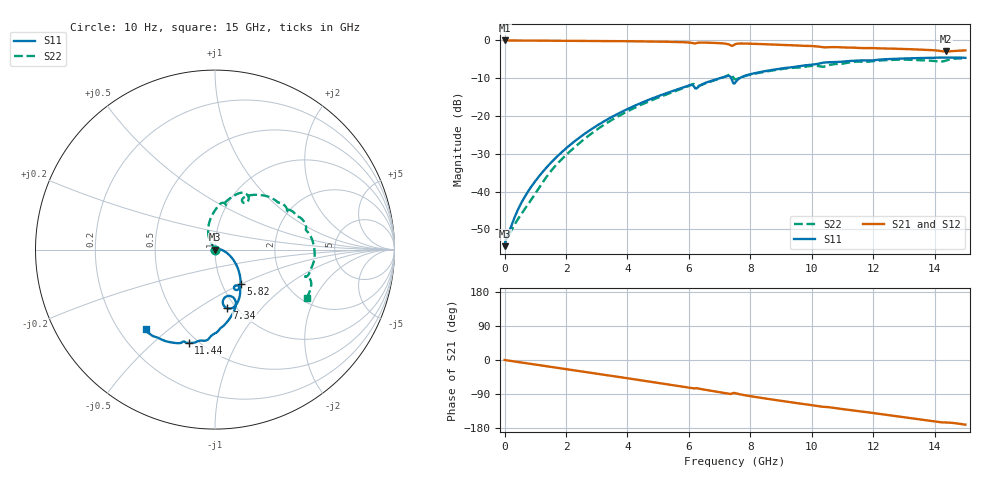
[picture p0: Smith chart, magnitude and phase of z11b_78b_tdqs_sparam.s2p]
![Disclaimer] This software code/ model/ data and all associated documentation, comments
!    or other information (collectively "Software") is provided
!    "AS IS" without warranty of any kind. MICRON TECHNOLOGY, INC.
!   ("MTI") EXPRESSLY DISCLAIMS ALL WARRANTIES EXPRESS OR IMPLIED,
!    INCLUDING BUT NOT LIMITED TO, NONINFRINGEMENT OF THIRD PARTY
!   RIGHTS, AND ANY IMPLIED WARRANTIES OF MERCHANTABILITY OR FITNESS
!    FOR ANY PARTICULAR PURPOSE. MTI DOES NOT WARRANT THAT THE
!    SOFTWARE WILL MEET YOUR REQUIREMENTS, OR THAT THE OPERATION OF
!    THE SOFTWARE WILL BE UNINTERRUPTED OR ERROR-FREE. FURTHERMORE,
!    MTI DOES NOT MAKE ANY REPRESENTATIONS REGARDING THE USE OR THE
!    RESULTS OF THE USE OF THE SOFTWARE IN TERMS OF ITS CORRECTNESS,
!    ACCURACY, RELIABILITY, OR OTHERWISE. THE ENTIRE RISK ARISING OUT
!    OF USE OR PERFORMANCE OF THE SOFTWARE REMAINS WITH YOU. IN NO
!    EVENT SHALL MTI, ITS AFFILIATED COMPANIES OR THEIR SUPPLIERS BE
!    LIABLE FOR ANY DIRECT, INDIRECT, CONSEQUENTIAL, INCIDENTAL, OR
!    SPECIAL DAMAGES (INCLUDING, WITHOUT LIMITATION, DAMAGES FOR LOSS
!    OF PROFITS, BUSINESS INTERRUPTION, OR LOSS OF INFORMATION)
!    ARISING OUT OF YOUR USE OF OR INABILITY TO USE THE SOFTWARE,
!    EVEN IF MTI HAS BEEN ADVISED OF THE POSSIBILITY OF SUCH DAMAGES.
!    Because some jurisdictions prohibit the exclusion or limitation
!    of liability for consequential or incidental damages, the above
!    limitation may not apply to you.
!    Copyright 2019 Micron Technology, Inc. All rights reserved.
! Single-ended  S-parameters
!NUMBER OF PORTS = 2
!  PORT#  PORT_NAME  NET_NAME
! PORT1:  TDQS-C.BGA.VDDQ_VSS TDQS-C
! PORT2:  TDQS-C.Z11B_DIE.VDDQ_VSS TDQS-C
# HZ S  RI R 5.000000e+001
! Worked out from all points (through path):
!   1701 points, 10 Hz to 15 GHz, reference 50 ohm
!   highest |S21| = -0.02 dB at 4.299 kHz (marker M1); lowest = -2.9 dB at 14.36 GHz (marker M2)
!   group delay of S21, straight-line fit = 32.2 ps
!   lowest |S11| = -54.5 dB at 10 Hz (marker M3), VSWR 1.00, Z = 50.2 + j6.76e-08 ohm
!   |S11| at or under -10 dB: start of sweep to 7.009 GHz; 7.378 GHz to 7.652 GHz (274.3 MHz wide, 3.65 % of centre)
!   |S22| runs from -54.5 to -4.8 dB; largest |S21 - S12| = 0
!   S11 on the Smith chart (normalised r, x): 10 Hz: 1.00, +0.00; 5.82 GHz: 1.22, -0.50; 7.34 GHz: 0.91, -0.67; 11.44 GHz: 0.45, -0.66; 15 GHz: 0.31, -0.42
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10  0.00189 6.73e-10  0.9981 -2.84e-09  0.9981 -2.84e-09  0.00189 6.8e-10
4298.66  0.00189 2.89e-07  0.9981 -1.22e-06  0.9981 -1.22e-06  0.00189 2.92e-07
5.84341e7  0.00231 0.000645  0.9974 -0.0128  0.9974 -0.0128  0.00227 0.000696
4.1e8  0.00449 0.00314  0.9923 -0.0873  0.9923 -0.0873  0.00186 0.00373
8.8e8  0.0108 0.00463  0.9766 -0.1842  0.9766 -0.1842  -0.000951 0.00789
1.61e9  0.0264 0.0024  0.934 -0.3289  0.934 -0.3289  -0.00963 0.0186
2.51e9  0.0536 -0.00984  0.8529 -0.4947  0.8529 -0.4947  -0.0235 0.0399
3.64e9  0.0938 -0.0459  0.707 -0.6772  0.707 -0.6772  -0.0378 0.0884
5.01e9  0.1341 -0.1251  0.4735 -0.8387  0.4735 -0.8387  -0.024 0.1739
5.82e9  0.1423 -0.1923  0.3119 -0.8939  0.3119 -0.8939  0.00954 0.2324
6.06e9  0.1314 -0.2205  0.2559 -0.8959  0.2559 -0.8959  0.0296 0.2553
6.26e9  0.1214 -0.1991  0.2467 -0.8912  0.2467 -0.8912  0.055 0.2427
6.98e9  0.1299 -0.2854  0.0842 -0.9167  0.0842 -0.9167  0.0949 0.2934
7.34e9  0.068 -0.3265  0.00495 -0.8674  0.00495 -0.8674  0.1654 0.3143
7.51e9  0.0933 -0.2612  0.04 -0.8902  0.04 -0.8902  0.1581 0.2613
8.11e9  0.1017 -0.3514  -0.1083 -0.8942  -0.1083 -0.8942  0.1949 0.3027
1.001e10  -0.0174 -0.4773  -0.4147 -0.7323  -0.4147 -0.7323  0.3901 0.2436
1.144e10  -0.1462 -0.5202  -0.5577 -0.5718  -0.5577 -0.5718  0.5026 0.1444
1.251e10  -0.2239 -0.5201  -0.6435 -0.4407  -0.6435 -0.4407  0.5496 0.0256
1.382e10  -0.3171 -0.4913  -0.7054 -0.2525  -0.7054 -0.2525  0.5238 -0.1346
1.436e10  -0.3534 -0.4768  -0.6887 -0.1859  -0.6887 -0.1859  0.5181 -0.1513
1.5e10  -0.3851 -0.4439  -0.7268 -0.1194  -0.7268 -0.1194  0.5102 -0.2676
